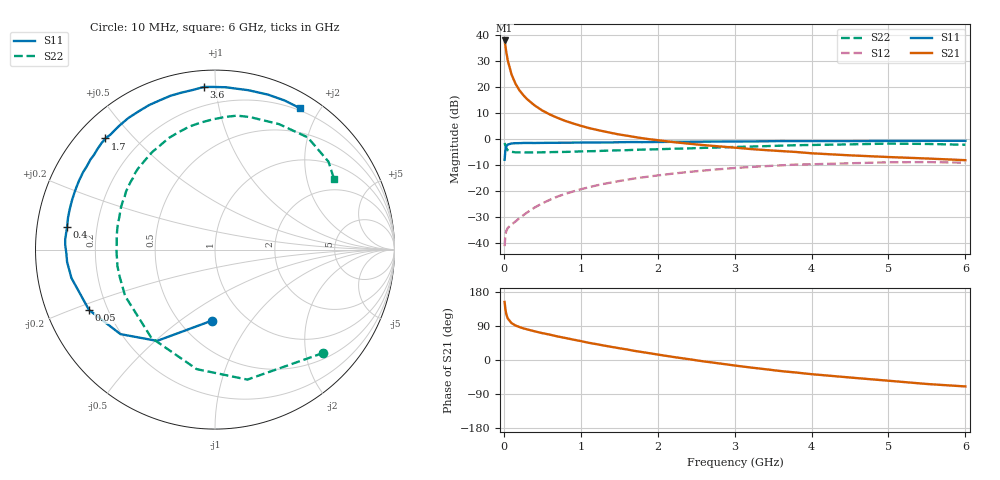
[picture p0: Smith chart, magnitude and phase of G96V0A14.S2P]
! SIEMENS Small Signal Semiconductors
! BFG235
! Si NPN RF Bipolar Junction Transistor in SOT223
! VCE = 6 V  IC = 140 mA
! Common Emitter S-Parameters:  July  1994
# GHz  S  MA  R  50
!  f  S11  S21  S12  S22
! GHz  MAG  ANG  MAG  ANG  MAG  ANG  MAG  ANG
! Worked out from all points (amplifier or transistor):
!   40 points, 10 MHz to 6 GHz, reference 50 ohm
!   highest |S21| = 37.8 dB at 10 MHz (marker M1)
!   |S21| within 3 dB of that: start of sweep to 24.84 MHz
!   unconditionally stable (mu >= 1): 463.8 MHz to 1.47 GHz
!   at 200 MHz: K = 0.80, MSG = 24.6 dB, |S12| = -30.5 dB
!   at 1.5 GHz: K = 1.00, MSG = 8.9 dB, |S12| = -16.2 dB
!   at 6 GHz: K = 0.89, MSG = 0.5 dB, |S12| = -9.1 dB
!   S11 on the Smith chart (normalised r, x): 10 MHz: 0.71, -0.66; 50 MHz: 0.13, -0.22; 400 MHz: 0.09, +0.08; 1.7 GHz: 0.08, +0.42; 3.6 GHz: 0.09, +0.93; 6 GHz: 0.17, +1.76
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0.01  0.3967 -92.7  77.69 153.2  0.0087 63.4  0.8343 -43.6
0.02  0.6024 -122.4  61.67 134.4  0.0142 49.3  0.7464 -76.0
0.03  0.7065 -138.2  48.69 122.5  0.0167 41.5  0.6738 -98.7
0.05  0.7783 -154.4  32.59 109.7  0.0194 34.2  0.6061 -125.8
0.1  0.8154 -168.8  17.27 97.4  0.0227 37.5  0.5637 -152.7
0.15  0.8269 -175.2  11.6 91.2  0.0258 43.2  0.5521 -164.0
0.2  0.8285 -178.6  8.686 87.2  0.0299 47.5  0.5514 -170.4
0.25  0.8348 178.3  6.997 83.7  0.0339 51.0  0.5484 -174.7
0.3  0.8366 176.1  5.837 81.0  0.0384 53.7  0.5488 -178.4
0.4  0.8337 171.3  4.394 75.7  0.048 56.7  0.5484 176.5
0.5  0.8378 167.8  3.507 70.9  0.0578 58.1  0.5526 172.3
0.6  0.8401 164.7  2.931 66.8  0.0678 57.8  0.5563 168.3
0.7  0.8427 161.1  2.526 62.1  0.0783 57.6  0.5606 164.9
0.9  0.8471 155.5  1.978 53.9  0.0976 54.8  0.5678 158.7
1.1  0.8521 149.5  1.623 45.5  0.1175 51.6  0.5795 152.6
1.7  0.8694 134.6  1.088 24.0  0.1736 39.5  0.6161 136.3
2.2  0.8778 123.4  0.869 8.1  0.2153 28.4  0.6465 122.7
3.2  0.8942 102.1  0.64 -19.6  0.2879 5.2  0.7112 96.8
3.6  0.9084 93.9  0.584 -29.2  0.3103 -4.7  0.7406 85.8
4.5  0.9074 78.1  0.483 -46.2  0.3399 -24.5  0.785 62.9
5.5  0.917 64.9  0.42 -63.3  0.3585 -46.5  0.7997 37.7
6  0.9191 58.8  0.39 -69.8  0.3489 -54.7  0.7704 30.5
